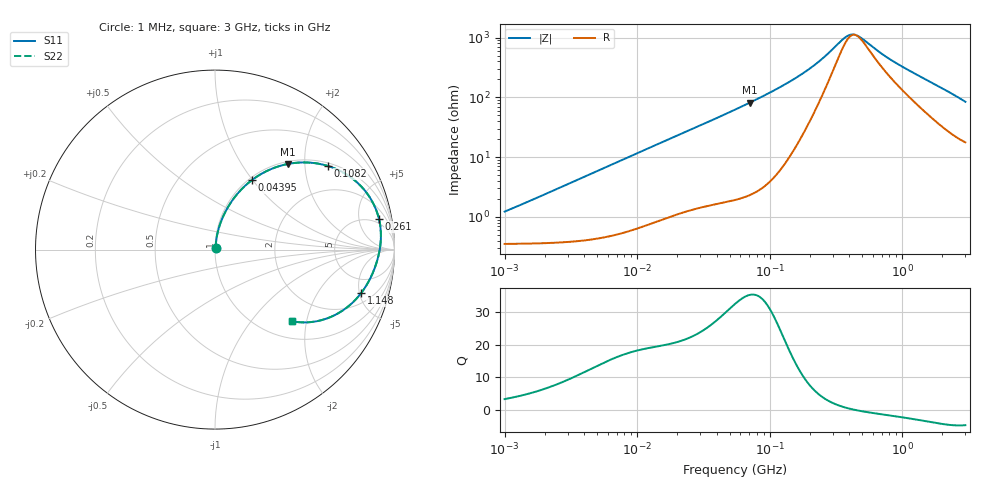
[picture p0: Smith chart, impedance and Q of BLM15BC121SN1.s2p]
! BLM15BC121SN1
# Hz S RI R 50
!Freq.(Hz) S11(Real) S11(Imag) S21(Real) S21(Imag) S12(Real) S12(Imag) S22(Real) S22(Imag)
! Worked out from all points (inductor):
!   401 points, 1 MHz to 3 GHz, reference 50 ohm
!   read as one part in series: L = 187 nH near 1.041 MHz
!   highest Q = 35.3 at 71.05 MHz (marker M1), where L = 184 nH
!   self-resonance near 442.3 MHz
!   S11 on the Smith chart (normalised r, x): 1 MHz: 1.01, +0.02; 43.95 MHz: 1.03, +1.00; 108.2 MHz: 1.09, +2.63; 261 MHz: 4, +9; 1.148 GHz: 2.96, -5.17; 3 GHz: 1.35, -1.65
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1000000  0.00366 0.0117  0.9963 -0.0117  0.9963 -0.0117  0.00366 0.0117
3823119  0.00597 0.0444  0.994 -0.0444  0.994 -0.0444  0.00597 0.0444
7858845  0.0136 0.09  0.9864 -0.09  0.9864 -0.09  0.0136 0.09
1.461624e7  0.0355 0.1612  0.9645 -0.1612  0.9645 -0.1612  0.0355 0.1612
2.718395e7  0.0971 0.2751  0.9029 -0.2751  0.9029 -0.2751  0.0971 0.2751
4.394807e7  0.2069 0.3882  0.7931 -0.3882  0.7931 -0.3882  0.2069 0.3882
5.477226e7  0.2861 0.4368  0.7139 -0.4368  0.7139 -0.4368  0.2861 0.4368
7.105049e7  0.4049 0.4769  0.5951 -0.4769  0.5951 -0.4769  0.4049 0.4769
8.854986e7  0.5209 0.485  0.4791 -0.485  0.4791 -0.485  0.5209 0.485
1.081723e8  0.6289 0.4658  0.3711 -0.4658  0.3711 -0.4658  0.6289 0.4658
1.520175e8  0.7881 0.3775  0.2119 -0.3775  0.2119 -0.3775  0.7881 0.3775
2.094008e8  0.8822 0.2564  0.1178 -0.2564  0.1178 -0.2564  0.8822 0.2564
2.609752e8  0.9135 0.171  0.0865 -0.171  0.0865 -0.171  0.9135 0.171
3.667557e8  0.9239 0.0546  0.0761 -0.0546  0.0761 -0.0546  0.9239 0.0546
3.973271e8  0.9219 0.0305  0.0781 -0.0305  0.0781 -0.0305  0.9219 0.0305
4.219165e8  0.9198 0.0132  0.0802 -0.0132  0.0802 -0.0132  0.9198 0.0132
4.853736e8  0.9127 -0.0253  0.0873 0.0253  0.0873 0.0253  0.9127 -0.0253
8.005644e8  0.8694 -0.1514  0.1306 0.1514  0.1306 0.1514  0.8694 -0.1514
1.147801e9  0.8131 -0.2437  0.1869 0.2437  0.1869 0.2437  0.8131 -0.2437
1.818868e9  0.6799 -0.3584  0.3201 0.3584  0.3201 0.3584  0.6799 -0.3584
2.359433e9  0.5621 -0.4  0.4379 0.4  0.4379 0.4  0.5621 -0.4
3e9  0.4311 -0.3995  0.5689 0.3995  0.5689 0.3995  0.4311 -0.3995
